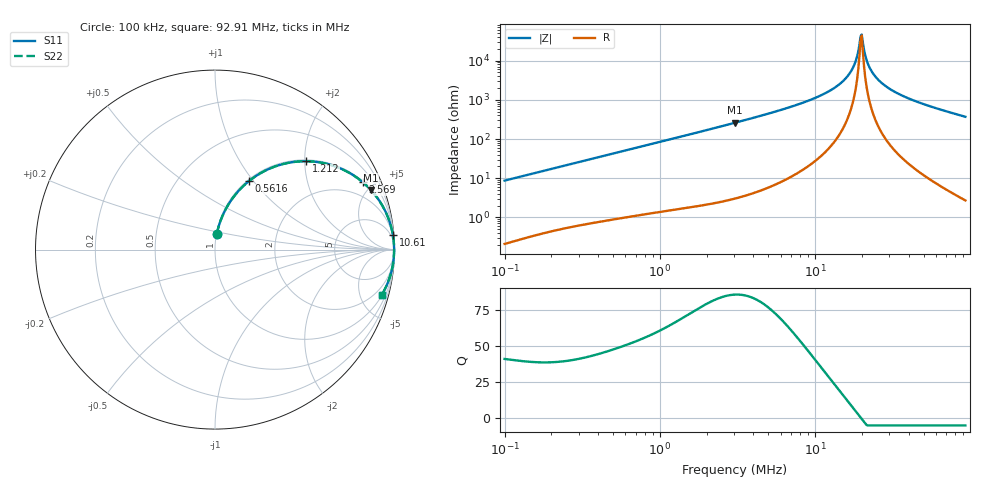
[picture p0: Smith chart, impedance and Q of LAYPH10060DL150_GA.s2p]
! LAYPH10060DL150_GA  S-PARAMETER MODEL  ( General Type )
! Model Generated by TAIYO YUDEN Corporation (http://www.ty-top.com)
! Version 3.0
! TAIYO YUDEN Control No. 180828NI43SB-FBB
! Copyright(c) 2017 TAIYO YUDEN CO.,LTD. All Rights Reserved.
! Product Description (link to TY-COMPAS)
! https://ds.yuden.co.jp/TYCOMPAS/or/detail?pn=LAYPH10060DL150MGA&u=M
! Products Name : Inductors
! Characteristics :
!  Inductance : 15 uH , SRF(min) : -Hz , DC Resistance(max) : 0.037 Ohm
!  Rated Current : Saturation :3.7 A , Temp Rise : 2.5 A (25 degC)
!  Case Size : 10.1 x 10.0 / 0.398 x 0.394 [mm/inch] , Thickness : 6 / 0.236 [mm/inch]
!  (Conditions: Temperature = 25 degC , DC Bias Current/Voltage = 0A / 0V)
! External Node Assignments :
!  1  o---GGG---o  2
! GND o---------o GND
! Frequency Range : 0.1MHz  -  92.907885MHz  [ 402 STEP ]
# MHz S RI R 50
! Freq[MHz].  S11 Real  S11 Imag  S21 Real  S21 Imag  S12 Real  S12 Imag  S22 Real  S22 Imag
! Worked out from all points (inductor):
!   401 points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, 100 kHz to 92.91 MHz, reference 50 ohm
!   read as one part in series: L = 13.8 uH near 103.5 kHz
!   highest Q = 85.9 at 3.048 MHz (marker M1), where L = 13.6 uH
!   self-resonance near 19.63 MHz
!   S11 on the Smith chart (normalised r, x): 100 kHz: 1.00, +0.17; 561.6 kHz: 1.02, +0.95; 1.212 MHz: 1.03, +2.03; 2.569 MHz: 1.05, +4.35; 10.61 MHz: 2, +25; 92.91 MHz: 1.05, -7.38
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0.1  0.00954 0.0858  0.9905 -0.0858  0.9905 -0.0858  0.00954 0.0858
0.314158  0.0718 0.2464  0.9282 -0.2464  0.9282 -0.2464  0.0718 0.2464
0.561608  0.1882 0.3809  0.8118 -0.3809  0.8118 -0.3809  0.1882 0.3809
0.986956  0.4087 0.4834  0.5913 -0.4834  0.5913 -0.4834  0.4087 0.4834
1.211544  0.5082 0.4924  0.4918 -0.4924  0.4918 -0.4924  0.5082 0.4924
2.56936  0.8227 0.376  0.1773 -0.376  0.1773 -0.376  0.8227 0.376
3.048079  0.8681 0.3326  0.1319 -0.3326  0.1319 -0.3326  0.8681 0.3326
3.100605  0.8721 0.3282  0.1279 -0.3282  0.1279 -0.3282  0.8721 0.3282
9.575801  0.9886 0.095  0.0114 -0.095  0.0114 -0.095  0.9886 0.095
10.60952  0.9914 0.0801  0.00864 -0.0801  0.00864 -0.0801  0.9914 0.0801
13.70875  0.9958 0.0456  0.00417 -0.0456  0.00417 -0.0456  0.9958 0.0456
16.26294  0.9974 0.0242  0.00264 -0.0242  0.00264 -0.0242  0.9974 0.0242
17.71331  0.9978 0.0137  0.00222 -0.0137  0.00222 -0.0137  0.9978 0.0137
18.32906  0.9979 0.00958  0.00212 -0.00958  0.00212 -0.00958  0.9979 0.00958
19.29303  0.998 0.00339  0.00203 -0.00339  0.00203 -0.00339  0.998 0.00339
19.96369  0.998 -0.000741  0.00202 0.000741  0.00202 0.000741  0.998 -0.000741
20.30771  0.998 -0.0028  0.00203 0.0028  0.00203 0.0028  0.998 -0.0028
21.7441  0.9979 -0.0111  0.00213 0.0111  0.00213 0.0111  0.9979 -0.0111
23.28209  0.9976 -0.0194  0.00238 0.0194  0.00238 0.0194  0.9976 -0.0194
30.08319  0.9953 -0.0516  0.00466 0.0516  0.00466 0.0516  0.9953 -0.0516
46.90804  0.9844 -0.1156  0.0156 0.1156  0.0156 0.1156  0.9844 -0.1156
92.90788  0.93 -0.2515  0.07 0.2515  0.07 0.2515  0.93 -0.2515
